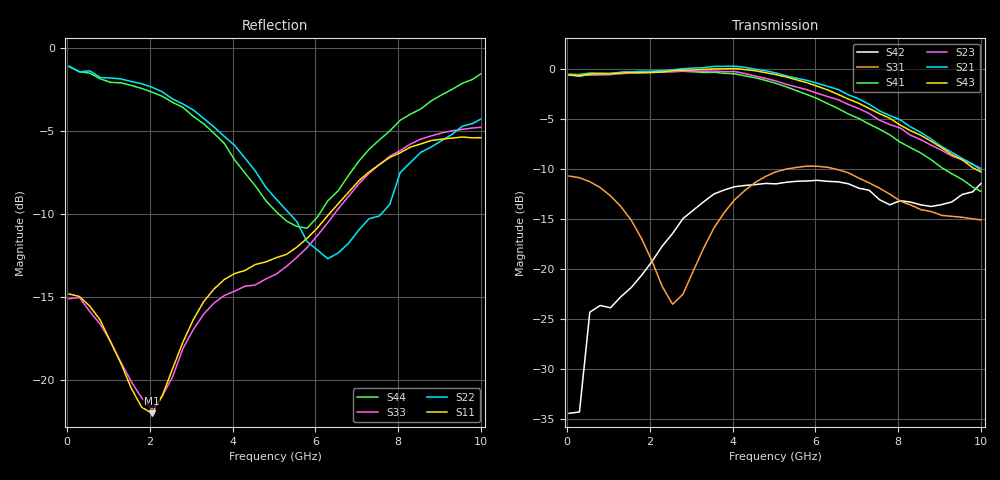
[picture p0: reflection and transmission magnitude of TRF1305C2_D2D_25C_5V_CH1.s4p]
! Created Mon Jun 30 19:23:07 2025
# hz S ma R 50
! PORT[1] = INP
! PORT[2] = OUTM
! PORT[3] = INM
! PORT[4] = OUTP
! 4 Port Network Data from SP1.SP block
! freq  magS11  angS11  magS12  angS12  magS13  angS13  magS14  angS14
!  magS21  angS21  magS22  angS22  magS23  angS23  magS24  angS24
!  magS31  angS31  magS32  angS32  magS33  angS33  magS34  angS34
!  magS41  angS41  magS42  angS42  magS43  angS43  magS44  angS44
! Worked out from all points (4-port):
!   41 points, 50 MHz to 10 GHz, reference 50 ohm
!   strongest paths, dB at 50 MHz, 2.55 GHz, 5.05 GHz, 7.55 GHz, 10 GHz:
!     S43: -0.6, -0.2, -0.5, -4.4, -10.3
!     S21: -0.6, -0.1, -0.4, -4.2, -10.1
!     S23: -0.6, -0.3, -1.2, -5.1, -9.9
!     S41: -0.5, -0.2, -1.4, -6.0, -12.2
!     S31: -10.7, -23.5, -10.3, -11.9, -15.1
!     S42: -34.4, -16.4, -11.5, -13.1, -11.4
!   lowest |S11| = -22.0 dB at 2.05 GHz (marker M1), VSWR 1.17, Z = 58.5 + j1.67 ohm
!   |S11| at or under -10 dB: start of sweep to 6.333 GHz
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5e7  0.1817 -1.8  0.003065 56.6  0.2873 -1.9  0.002104 159.7
     0.9381 178.2  0.8803 -179.6  0.9317 -1.2  0.009247 159.3
     0.292 -2.5  0.003559 138.4  0.1758 -0.6  0.005131 33.7
     0.9426 -1.3  0.01898 138.1  0.9352 178.5  0.8773 -179.7
5.5e8  0.167 -14.2  0.03296 57.6  0.2668 -22.8  0.02575 62.3
       0.9407 158.8  0.8522 174.6  0.9347 -20.6  0.061 57.4
       0.2736 -23.4  0.02587 58.7  0.1609 -13.4  0.03566 53.3
       0.9562 -19.3  0.06083 56.9  0.9451 159.4  0.8387 176.5
2.05e9  0.07951 10.3  0.05828 11.1  0.1094 -96.3  0.03681 -5.3
        0.9764 96.2  0.7613 171.0  0.9629 -79.5  0.1138 -32.8
        0.11 -100.6  0.0357 -9.1  0.0819 4.5  0.06038 12.5
        0.969 -75.8  0.109 -32.0  0.9631 99.5  0.736 -178.6
4.05e9  0.2094 18.6  0.08711 -35.0  0.2122 73.4  0.03717 -70.3
        1.035 11.6  0.5084 172.4  0.9733 -163.8  0.2637 -59.2
        0.2222 70.7  0.03622 -78.6  0.1852 15.2  0.09006 -29.0
        0.9484 -158.0  0.2582 -60.1  1.007 18.6  0.4598 -162.3
6.05e9  0.2871 7.6  0.105 -85.4  0.3273 12.1  0.01274 -126.8
        0.8494 -77.0  0.2463 -164.5  0.7572 103.8  0.2911 -92.1
        0.3267 8.2  0.008637 -164.2  0.2724 9.6  0.1064 -75.9
        0.7121 113.0  0.2778 -91.9  0.8212 -65.8  0.3096 -123.3
6.55e9  0.3392 2.4  0.1105 -97.7  0.3153 -0.2  0.007539 -72.8
        0.791 -97.9  0.2413 -139.6  0.7034 81.5  0.2831 -92.5
        0.314 -4.1  0.001721 -11.1  0.3274 4.0  0.1068 -86.4
        0.6354 90.6  0.2732 -92.4  0.7478 -85.8  0.3712 -106.5
1e10  0.5365 -77.1  0.1086 178.3  0.1835 -36.6  0.04554 -96.5
      0.3128 142.5  0.6105 -108.2  0.3197 -56.0  0.2653 -45.9
      0.1763 -34.3  0.04469 -102.0  0.5765 -81.7  0.1051 -158.0
      0.2449 -39.3  0.2678 -43.1  0.3064 166.3  0.8353 -73.0
